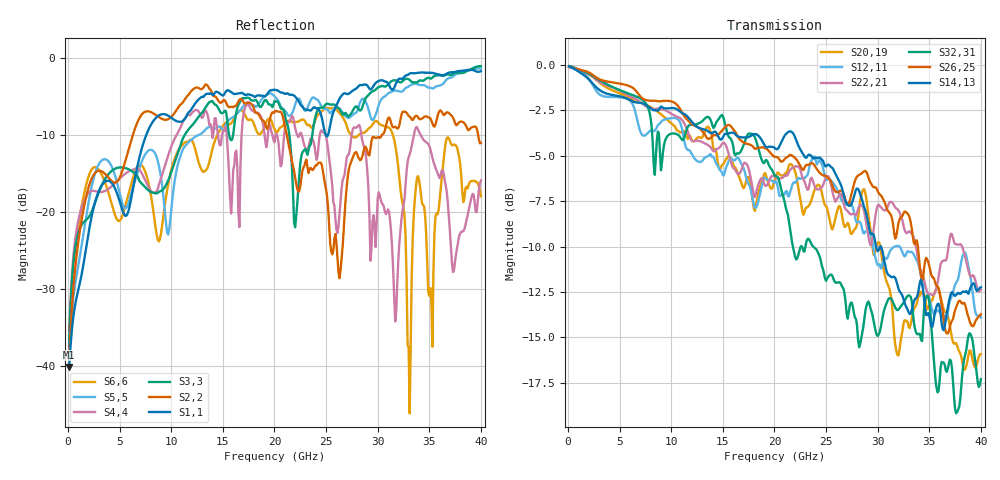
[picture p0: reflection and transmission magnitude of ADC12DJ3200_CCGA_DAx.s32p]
! Touchstone file
! Texas Instruments 4/21/2021
! ADC12DJ3200QML-SP
! Package-type  CCGA [BGA]
! pins/pkg drawing  196-pin NWE
! CCGA Ceramic Package with columns (ceramic column grid array)
! High-speed serialized data output for channel A, lane 0-7
# GHZ S MA R 50.000000
! Port[1] = DA0N_BGA_F14
! Port[2] = DA0N_DIE_22
! Port[3] = DA0P_BGA_E14
! Port[4] = DA0P_DIE_21
! Port[5] = DA1N_BGA_D14
! Port[6] = DA1N_DIE_24
! Port[7] = DA1P_BGA_C14
! Port[8] = DA1P_DIE_23
! Port[9] = DA2N_BGA_A13
! Port[10] = DA2N_DIE_26
! Port[11] = DA2P_BGA_A12
! Port[12] = DA2P_DIE_25
! Port[13] = DA3N_BGA_A11
! Port[14] = DA3N_DIE_28
! Port[15] = DA3P_BGA_A10
! Port[16] = DA3P_DIE_27
! Port[17] = DA4N_BGA_F13
! Port[18] = DA4N_DIE_30
! Port[19] = DA4P_BGA_E13
! Port[20] = DA4P_DIE_29
! Port[21] = DA5N_BGA_D13
! Port[22] = DA5N_DIE_32
! Port[23] = DA5P_BGA_C13
! Port[24] = DA5P_DIE_31
! Port[25] = DA6N_BGA_B13
! Port[26] = DA6N_DIE_34
! Port[27] = DA6P_BGA_B12
! Port[28] = DA6P_DIE_33
! Port[29] = DA7N_BGA_B11
! Port[30] = DA7N_DIE_36
! Port[31] = DA7P_BGA_B10
! Port[32] = DA7P_DIE_35
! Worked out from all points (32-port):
!   400 points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, 100 MHz to 40 GHz, reference 50 ohm
!   strongest paths, dB at 100 MHz, 10.1 GHz, 20.1 GHz, 30.1 GHz, 40 GHz:
!     S14,13: -0.1, -2.4, -4.6, -10.2, -12.2
!     S26,25: -0.1, -2.0, -5.1, -7.1, -13.7
!     S32,31: -0.1, -3.8, -6.1, -14.8, -17.3
!     S22,21: -0.1, -2.7, -6.2, -7.7, -12.4
!     S12,11: -0.1, -2.9, -6.4, -11.0, -13.9
!     S20,19: -0.1, -3.3, -6.2, -9.7, -15.9
!   lowest |S11| = -40.2 dB at 100 MHz (marker M1), VSWR 1.02, Z = 50.9 + j0.454 ohm
!   |S11| at or under -10 dB: start of sweep to 7.559 GHz; 24.99 GHz to 25.18 GHz (183.1 MHz wide, 0.73 % of centre)
